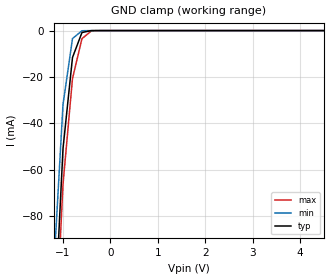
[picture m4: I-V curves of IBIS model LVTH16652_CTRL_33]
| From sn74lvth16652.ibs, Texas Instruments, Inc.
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|   Model LVTH16652 Input_CTRL_33
[Model]   LVTH16652_CTRL_33
Model_type  Input
Polarity   Inverting
Vinl = 0.8V
Vinh = 2.0V
| variable   typ   min   max
C_comp   4pf   NA   NA
[Temperature Range]   40   -25   100
| Ambient temperature   25   -40   85
[Voltage range]   3.3   3.0   3.6
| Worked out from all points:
|   GND clamp passes 1 mA (typ) near -0.60 V on its own axis
[GND Clamp]
|   Voltage   I(typ)   I(min)   I(max)
-5V       -2.436A    -2.821A    -2.132A
-1.2V     -134.3mA   -104.7mA   -149.8mA
-1V       -50.88mA   -31.86mA   -66.32mA
-800mV    -11.63mA   -3.438mA   -20.67mA
-600mV    -827uA     -69.69uA   -3.479mA
-400mV    -3.023uA   -83.2nA    -129.8uA
-200mV    -2.389nA   -22.83nA   -385.1nA
5V        66.02pA    605.7nA    418.1pA
